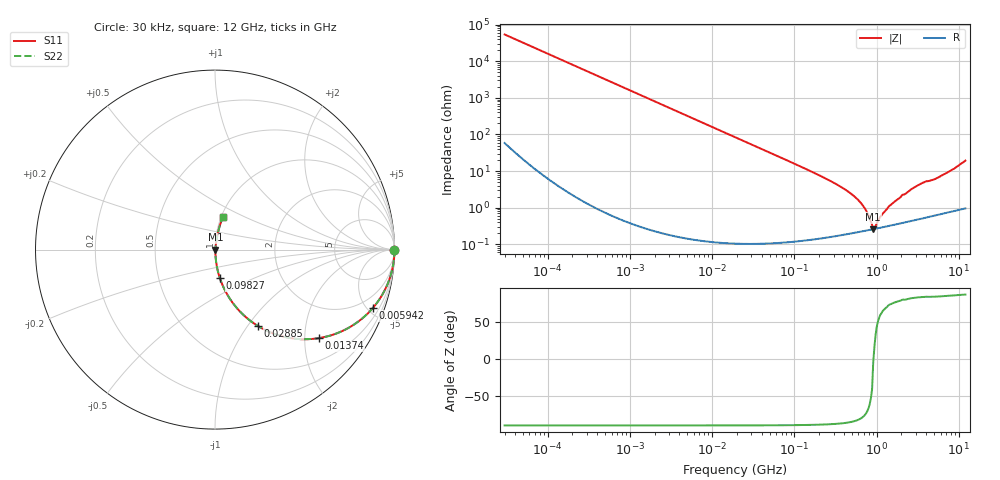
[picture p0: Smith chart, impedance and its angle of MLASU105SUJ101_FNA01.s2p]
! MLASU105SUJ101_FNA01  S-PARAMETER MODEL  ( General Type )
! Model Generated by TAIYO YUDEN Corporation (http://www.ty-top.com)
! Version 4.0
! TAIYO YUDEN Control No. 131101
! Copyright(c) 2003 TAIYO YUDEN CO.,LTD. All Rights Reserved.
! Product Description (link to TY-COMPAS)
! https://ds.yuden.co.jp/TYCOMPAS/or/detail?pn=MLASU105SUJ101JFNA01&u=M
! Products Name : Multilayer Ceramic Capacitors
! Characteristics :
!  Capacitance : 100 pF , Rated Voltage : 50V , TCC : UJ / U2J
!  Case Size : 1.0 x 0.5 / 0.039 x 0.02 [mm/inch] , Thickness : 0.5 / 0.02 [mm/inch]
!  (Conditions: Temperature = 25 degC , DC Bias Current/Voltage = 0A / 0V)
! External Node Assignments :
!  1  o---| |---o  2
! GND o---------o GND
! Frequency Range : 0.03MHz  -  12000MHz  [ 401 STEP ]
# MHz S RI R 50
! Freq[MHz].  S11 Real  S11 Imag  S21 Real  S21 Imag  S12 Real  S12 Imag  S22 Real  S22 Imag
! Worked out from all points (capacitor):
!   401 points, 30 kHz to 12 GHz, reference 50 ohm
!   read as one part in series: C = 98.7 pF near 32 kHz
!   lowest |Z| = 260 mohm at 909.4 MHz (marker M1)
!   series resonance near 915.5 MHz, so ESL is about 310 pH
!   S11 on the Smith chart (normalised r, x): 30 kHz: open; 5.942 MHz: 1.00, -5.43; 13.74 MHz: 1.00, -2.35; 28.85 MHz: 1.00, -1.12; 98.27 MHz: 1.00, -0.32; 12 GHz: 1.02, +0.39
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0.03  1 -0.00186  5.49e-06 0.00186  5.49e-06 0.00186  1 -0.00186
0.260295  0.9997 -0.0161  0.000264 0.0161  0.000264 0.0161  0.9997 -0.0161
2.258455  0.9807 -0.1373  0.0193 0.1373  0.0193 0.1373  0.9807 -0.1373
5.942454  0.8803 -0.3243  0.1197 0.3243  0.1197 0.3243  0.8803 -0.3243
9.037177  0.7609 -0.4262  0.2391 0.4262  0.2391 0.4262  0.7609 -0.4262
13.74358  0.5791 -0.4932  0.4209 0.4932  0.4209 0.4932  0.5791 -0.4932
18.97367  0.4193 -0.4928  0.5807 0.4928  0.5807 0.4928  0.4193 -0.4928
28.85481  0.2381 -0.425  0.7619 0.425  0.7619 0.425  0.2381 -0.425
49.92358  0.0948 -0.2913  0.9052 0.2913  0.9052 0.2913  0.0948 -0.2913
98.2684  0.0268 -0.1578  0.9732 0.1578  0.9732 0.1578  0.0268 -0.1578
164.6252  0.0102 -0.0939  0.9898 0.0939  0.9898 0.0939  0.0102 -0.0939
345.6326  0.00334 -0.0401  0.9967 0.0401  0.9967 0.0401  0.00334 -0.0401
542.8588  0.00246 -0.0197  0.9975 0.0197  0.9975 0.0197  0.00246 -0.0197
702.6322  0.00241 -0.0101  0.9976 0.0101  0.9976 0.0101  0.00241 -0.0101
909.4299  0.00258 -0.000187  0.9974 0.000187  0.9974 0.000187  0.00258 -0.000187
970.0175  0.00266 0.00166  0.9973 -0.00166  0.9973 -0.00166  0.00266 0.00166
1139.739  0.0029 0.00528  0.9971 -0.00528  0.9971 -0.00528  0.0029 0.00528
1428.372  0.00331 0.0107  0.9967 -0.0107  0.9967 -0.0107  0.00331 0.0107
2903.719  0.0058 0.0355  0.9942 -0.0355  0.9942 -0.0355  0.0058 0.0355
3758.338  0.00754 0.0484  0.9925 -0.0484  0.9925 -0.0484  0.00754 0.0484
5534.236  0.0105 0.0646  0.9895 -0.0646  0.9895 -0.0646  0.0105 0.0646
12000  0.0445 0.1828  0.9555 -0.1828  0.9555 -0.1828  0.0445 0.1828
